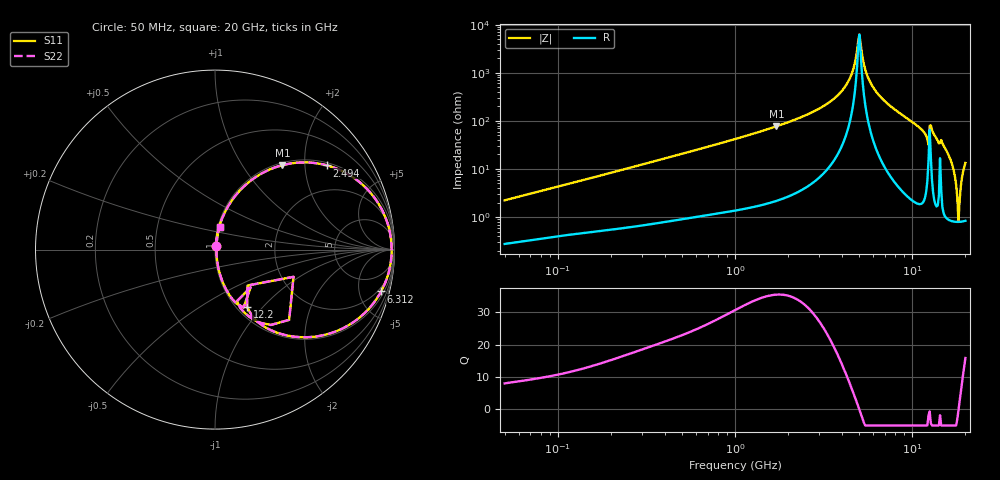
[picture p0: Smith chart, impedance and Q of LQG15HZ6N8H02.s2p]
!Murata Part Number: LQG15HZ6N8H02
!These Parameters are Measured in Series Mode Connection
!  o--[Z]--o
!Port1  Port2
!  o-------o
!Freq. Start=50[MHz] Stop=20[GHz], 401[Steps]
# Hz S RI R 50
!Freq.(Hz) S11(Real) S11(Imag) S21(Real) S21(Imag) S12(Real) S12(Imag) S22(Real) S22(Imag)
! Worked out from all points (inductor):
!   401 points, 50 MHz to 20 GHz, reference 50 ohm
!   read as one part in series: L = 6.96 nH near 51.52 MHz
!   highest Q = 35.4 at 1.715 GHz (marker M1), where L = 7.15 nH
!   self-resonance near 4.967 GHz
!   S11 on the Smith chart (normalised r, x): 50 MHz: 1.01, +0.04; 2.494 GHz: 1.08, +2.60; 6.312 GHz: 1.49, -7.80; 12.2 GHz: 1.11, -0.82; 20 GHz: 1.02, +0.27
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5e7  0.00325 0.022  0.9968 -0.022  0.9968 -0.022  0.00325 0.022
1.364002e8  0.00786 0.0569  0.9921 -0.0569  0.9921 -0.0569  0.00786 0.0569
3.721004e8  0.03 0.1477  0.97 -0.1477  0.97 -0.1477  0.03 0.1477
1e9  0.1567 0.3476  0.8433 -0.3476  0.8433 -0.3476  0.1567 0.3476
1.714689e9  0.376 0.4705  0.624 -0.4705  0.624 -0.4705  0.376 0.4705
2.493527e9  0.624 0.4691  0.376 -0.4691  0.376 -0.4691  0.624 0.4691
2.728004e9  0.6899 0.4462  0.3101 -0.4462  0.3101 -0.4462  0.6899 0.4462
4.149438e9  0.9458 0.1886  0.0542 -0.1886  0.0542 -0.1886  0.9458 0.1886
4.608136e9  0.9758 0.0895  0.0242 -0.0895  0.0242 -0.0895  0.9758 0.0895
5.041459e9  0.9843 -0.00179  0.0157 0.00179  0.0157 0.00179  0.9843 -0.00179
5.598765e9  0.9717 -0.1113  0.0283 0.1113  0.0283 0.1113  0.9717 -0.1113
6.311513e9  0.9258 -0.2329  0.0742 0.2329  0.0742 0.2329  0.9258 -0.2329
7.442007e9  0.8085 -0.3761  0.1915 0.3761  0.1915 0.3761  0.8085 -0.3761
1.034674e10  0.4322 -0.4838  0.5678 0.4838  0.5678 0.4838  0.4322 -0.4838
1.220001e10  0.1782 -0.3191  0.8218 0.3191  0.8218 0.3191  0.1782 -0.3191
1.314879e10  0.2553 -0.4086  0.7447 0.4086  0.7447 0.4086  0.2553 -0.4086
1.573793e10  0.0572 -0.2128  0.9428 0.2128  0.9428 0.2128  0.0572 -0.2128
1.696185e10  0.0202 -0.109  0.9798 0.109  0.9798 0.109  0.0202 -0.109
1.774144e10  0.00993 -0.0448  0.9901 0.0448  0.9901 0.0448  0.00993 -0.0448
1.828096e10  0.00789 -0.00151  0.9921 0.00151  0.9921 0.00151  0.00789 -0.00151
1.88369e10  0.00973 0.042  0.9903 -0.042  0.9903 -0.042  0.00973 0.042
2e10  0.0252 0.1284  0.9748 -0.1284  0.9748 -0.1284  0.0252 0.1284
